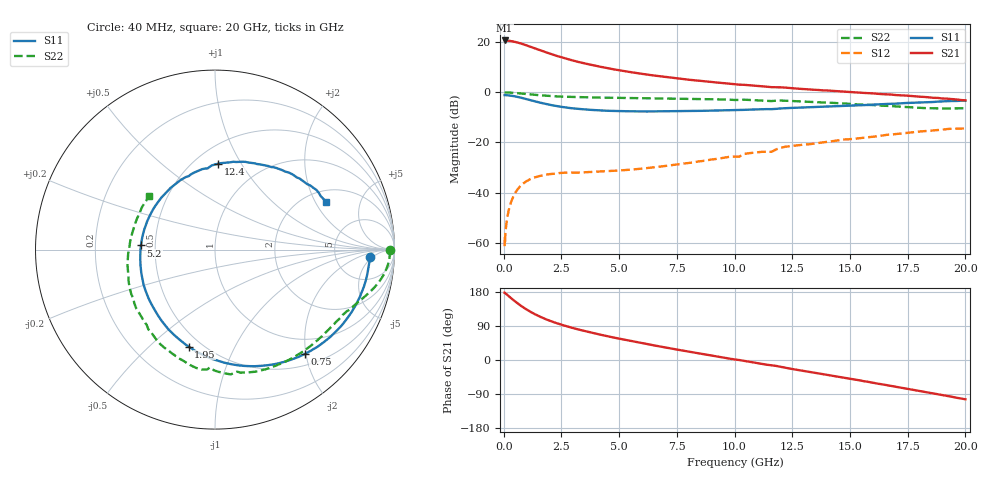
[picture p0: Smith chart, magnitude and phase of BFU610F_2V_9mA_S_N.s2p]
! Filename:  P:\Prog\Test\Noise\ATS_data\Testdata_Net\SplitFiles\BFU610_2W_A5_HighFreq_2V_9mA_D.s2p
! Date/Time: Wed 10/Aug/2011 16:56:11
! BFU610_2W_A5_HighFreq_2V_1mA_10mA_Bias6_R.s2p
! MDIF S-parameter v. bias file
! BFU610_2W_A5_HighFreq_2V_1mA_10mA
! Date/time Mon Aug 08 14:20:39 2011
! VAR V_out= 2.0003
! VAR I_out= 9.0000
! VAR V_in= 0.9283
! VAR I_in= 0.0838
! Device data file deembeded for feedlines and parallel
! Original file: \SplitFiles\BFU610_2W_A5_HighFreq_2V_9mA_R.s2p
! Feed-files: PR003V01_101208_Feed1.s2p, PR003V01_101208_Feed2.s2p
! Parallel-file: PR003V01_101208_Par.s2p
# MHz S MA R 50
!  Freq-MHz  S11-mag  S11-arg  S21-mag  S21-arg  S12-mag  S12-arg  S22-mag  S22-arg
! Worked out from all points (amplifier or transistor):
!   167 points, 40 MHz to 20 GHz, reference 50 ohm
!   highest |S21| = 20.5 dB at 40 MHz (marker M1)
!   |S21| within 3 dB of that: start of sweep to 1.308 GHz
!   unconditionally stable (mu >= 1): 2.281 GHz to end of sweep
!   at 550 MHz: K = 0.26, MSG = 29.6 dB, |S12| = -39.4 dB
!   at 4.2 GHz: K = 1.89, MAG = 15.4 dB, |S12| = -31.6 dB
!   at 20 GHz: K = 1.62, MAG = 1.0 dB, |S12| = -14.5 dB
!   lowest NFmin = 1.57 dB at 400 MHz
!   S11 on the Smith chart (normalised r, x): 40 MHz: 12, -4; 750 MHz: 0.70, -1.97; 1.95 GHz: 0.43, -0.67; 5.2 GHz: 0.42, +0.02; 12.4 GHz: 0.65, +0.80; 20 GHz: 2.51, +2.46
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40  0.8633 -2.7  10.53 177.8  0.0008582 80.6  0.9725 -0.2
50  0.863 -3.4  10.49 177.6  0.001268 58.8  0.9738 -0.5
60  0.8631 -4.1  10.53 176.5  0.001056 78.3  0.9744 -0.7
160  0.8579 -11.1  10.43 171.5  0.003237 82.8  0.9734 -2.6
400  0.8303 -27.4  10.08 159.1  0.007972 75.2  0.9606 -6.6
550  0.8056 -37.2  9.722 151.8  0.01067 69.7  0.948 -8.8
750  0.7669 -49.4  9.14 142.9  0.01377 63.0  0.9286 -11.5
1000  0.7166 -63.3  8.372 133.0  0.01692 55.8  0.9041 -14.3
1250  0.668 -75.9  7.621 124.2  0.01925 50.0  0.8811 -16.7
1600  0.6091 -91.6  6.681 113.6  0.02152 43.8  0.8548 -19.5
1950  0.5602 -105.2  5.877 104.7  0.02309 39.2  0.8342 -22.1
2250  0.5276 -115.5  5.287 98.0  0.02371 36.5  0.8181 -24.4
2600  0.4971 -126.4  4.726 91.3  0.0247 34.1  0.8028 -26.4
3400  0.4531 -147.1  3.784 78.1  0.02509 32.3  0.7838 -31.6
4200  0.4275 -164.7  3.151 66.7  0.02617 33.2  0.7702 -36.8
5200  0.4135 176.8  2.597 53.9  0.02778 36.5  0.758 -43.8
6800  0.41 151.9  2.034 35.3  0.03281 42.4  0.7411 -55.2
10200  0.435 109.5  1.392 -0.0  0.05159 48.0  0.6927 -80.3
12400  0.479 87.8  1.195 -22.8  0.08348 40.1  0.6617 -100.9
13400  0.4997 78.3  1.106 -32.9  0.09329 33.8  0.6294 -111.2
16800  0.5808 49.5  0.8853 -68.7  0.1423 10.5  0.5209 -155.7
20000  0.6731 23.4  0.6786 -103.7  0.1885 -21.8  0.4722 140.7
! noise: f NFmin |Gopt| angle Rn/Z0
400  1.567  0.408  2.487  0.4352
800  1.685  0.3717  6.914  0.4385
1250  1.824  0.3336  11.65  0.4398
1700  1.968  0.2975  16.07  0.4393
2150  2.117  0.2627  20.13  0.4376
2700  2.306  0.2212  24.48  0.4352
3600  2.634  0.1543  29.7  0.4336
4500  2.983  0.08889  29.89  0.4402
5800  3.524  0.02711  307.4  0.4764
8000  4.543  0.1455  264.5  0.656
